VAR_GLOBAL CONSTANT
	
	cSamplerate			: UDINT := 10000;													// Samplerate of input signal
	cOversamples 		: UDINT := 10;														// number of oversamples
	cWindowLength		: UDINT	:= 3200;													// internal buffer size with 50% overlapping
	cFFTLength			: UDINT	:= 4096;													// length of FFT for mag. spectrum	
	cFFTResult 			: UDINT := 2049;													// result of mag. spectrum (cFFTLength/2+1)
	cScalingType		: E_CM_ScalingType := E_CM_ScalingType.eCM_PeakAmplitude;			// scaling type
	
	// window analysis for spectrum 1
	// Hann window and explicit overlap of 50%, i.e. 1600.
	cWindowType1		: E_CM_WindowType 		:= E_CM_WindowType.eCM_HannWindow;			// window type for spectrum 1
	cWindowParameters1	: T_CM_WindowParameters := [0.0, 0.0, 0.0, 0.0, 0.0];				// window parameters for spectrum 1 - unused.
	cOverlap1			: UDINT	:= cWindowLength/2;											// size of overlap in signal analysis, see MAIN_CM: nOverlap1.
	cBufferLength1		: UDINT	:= cWindowLength - cOverlap1;  								// buffer size equals cWindowLength - cOverlap1
	
	// window analysis for spectrum 2
	// rectangular window and overlap inactive, i.e. 0.
	cWindowType2		: E_CM_WindowType 		:= E_CM_WindowType.eCM_RectangularWindow;	// window type for spectrum 2
	cWindowParameters2	: T_CM_WindowParameters := [0.0, 0.0, 0.0, 0.0, 0.0];				// window parameters for spectrum 2 - unused.
	cOverlap2			: UDINT	:= 0;														// size of overlap in signal analysis, see MAIN_CM: nOverlap2.
	cBufferLength2		: UDINT	:= cWindowLength - cOverlap2;  								// buffer size equals cWindowLength - cOverlap2

	// window analysis for spectrum 3
	// Bartlett window and explicit overlap of 50%, i.e. 1600.
	cWindowType3		: E_CM_WindowType 		:= E_CM_WindowType.eCM_BartlettWindow;		// window type for spectrum 3
	cWindowParameters3	: T_CM_WindowParameters := [0.0, 0.0, 0.0, 0.0, 0.0];				// window parameters for spectrum 3 - unused.
	cOverlap3			: UDINT	:= cWindowLength/2;											// size of overlap in signal analysis, see MAIN_CM: nOverlap3.
	cBufferLength3		: UDINT	:= cWindowLength - cOverlap3;  								// buffer size equals cWindowLength - cOverlap3
	
	
	// window analysis for spectrum 4
	// Hamming window and explicit overlap of 50%, i.e. 1600.
	cWindowType4		: E_CM_WindowType 		:= E_CM_WindowType.eCM_HammingWindow;		// window type for spectrum 4
	cWindowParameters4	: T_CM_WindowParameters := [0.0, 0.0, 0.0, 0.0, 0.0];				// window parameters for spectrum 4 - unused.
	cOverlap4			: UDINT	:= cWindowLength/2;											// size of overlap in signal analysis, see MAIN_CM: nOverlap4.
	cBufferLength4		: UDINT	:= cWindowLength - cOverlap4;  								// buffer size equals cWindowLength - cOverlap4
	
	// window analysis for spectrum 5
	// Kaiser-4 window and recommended overlap of 67%, i.e. 
	cWindowType5		: E_CM_WindowType 		:= E_CM_WindowType.eCM_KaiserWindow;		// window type for spectrum 5
	cWindowParameters5	: T_CM_WindowParameters := [4*PI, 0.0, 0.0, 0.0, 0.0];				// window parameters for spectrum 5 - unused.
	cOverlap5			: UDINT	:= 2143;													// size of overlap in signal analysis, see MAIN_CM: nOverlap5.
	cBufferLength5		: UDINT	:= cWindowLength - cOverlap5;  								// buffer size equals cWindowLength - cOverlap5

	// window analysis for spectrum 6
	// SFT5M window and recommended overlap of 76%, i.e. 2433. 
	cWindowType6		: E_CM_WindowType 		:= E_CM_WindowType.eCM_FlatTopWindow;		// window type for spectrum 6
	cWindowParameters6	: T_CM_WindowParameters 
							:= [0.209671, -0.407331, 0.281225, -0.092669, 0.0091036];		// window parameters for spectrum 6; SFT5M.
	cOverlap6			: UDINT	:= 2433;													// size of overlap in signal analysis, use MAIN_CM: nOverlap6.
	cBufferLength6		: UDINT	:= cWindowLength - cOverlap6;  								// buffer size equals cWindowLength - cOverlap6
	
END_VAR
